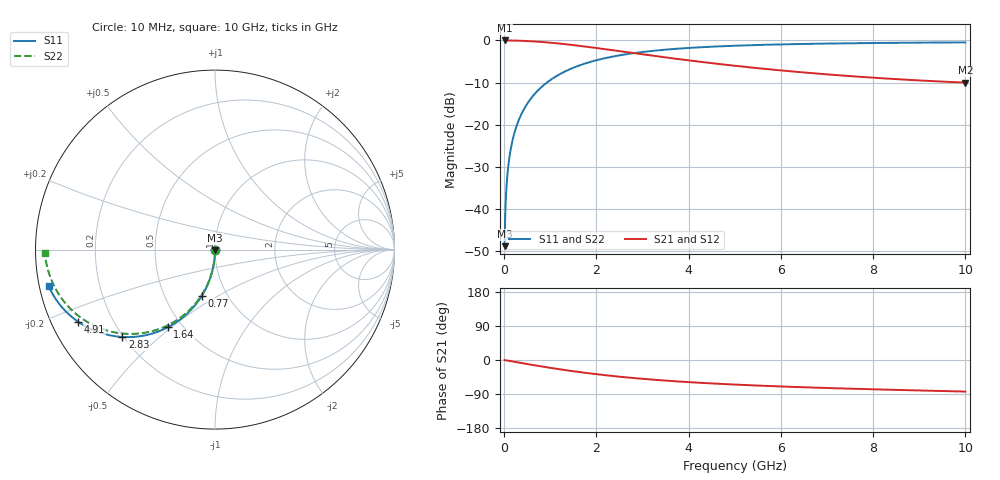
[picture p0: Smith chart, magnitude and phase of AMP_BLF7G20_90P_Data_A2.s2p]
! Created Tue May 08 13:45:06 2012
# ghz S ma R 50
! 2 Port Network Data from SP1.SP block
! freq  magS11  angS11  magS21  angS21  magS12  angS12  magS22  angS22
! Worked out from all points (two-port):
!   1000 points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, 10 MHz to 10 GHz, reference 50 ohm
!   highest |S21| = 0.00 dB at 10 MHz (marker M1); lowest = -10.0 dB at 10 GHz (marker M2)
!   |S21| within 3 dB of the highest: start of sweep to 2.804 GHz
!   lowest |S11| = -48.9 dB at 10 MHz (marker M3), VSWR 1.01, Z = 50 - j0.359 ohm
!   |S11| at or under -10 dB: start of sweep to 927.7 MHz
!   |S22| runs from -48.9 to -0.5 dB; largest |S21 - S12| = 0
!   S11 on the Smith chart (normalised r, x): 10 MHz: 1.00, -0.01; 770 MHz: 0.76, -0.42; 1.64 GHz: 0.42, -0.49; 2.83 GHz: 0.20, -0.38; 4.91 GHz: 0.08, -0.25; 10 GHz: 0.03, -0.11
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0.01  0.003594 -90.2  1 -0.2  1 -0.2  0.003594 -90.2
0.04  0.01438 -90.8  0.9999 -0.9  0.9999 -0.9  0.01438 -90.9
0.07  0.02516 -91.5  0.9997 -1.5  0.9997 -1.5  0.02516 -91.5
0.09  0.03234 -91.9  0.9995 -1.9  0.9995 -1.9  0.03234 -92.0
0.14  0.05028 -92.9  0.9987 -3.0  0.9987 -3.0  0.05028 -93.1
0.21  0.0753 -94.4  0.9971 -4.5  0.9971 -4.5  0.0753 -94.6
0.31  0.1108 -96.5  0.9938 -6.7  0.9938 -6.7  0.1108 -96.8
0.43  0.1528 -99.0  0.9882 -9.2  0.9882 -9.2  0.1528 -99.4
0.58  0.2041 -102.1  0.9789 -12.3  0.9789 -12.3  0.2041 -102.6
0.77  0.2667 -105.9  0.9637 -16.2  0.9637 -16.2  0.2667 -106.5
1.15  0.3817 -113.0  0.9243 -23.5  0.9243 -23.5  0.3817 -114.0
1.64  0.5068 -121.3  0.8621 -32.0  0.8621 -32.0  0.5067 -122.7
1.68  0.5158 -121.9  0.8567 -32.6  0.8567 -32.6  0.5158 -123.3
2.21  0.6197 -129.5  0.7848 -40.4  0.7848 -40.4  0.6197 -131.3
2.83  0.7093 -136.7  0.7048 -47.9  0.7048 -47.9  0.7093 -139.0
3.34  0.7634 -141.5  0.6459 -52.9  0.6459 -52.9  0.7634 -144.3
4.08  0.8197 -147.2  0.5727 -59.0  0.5727 -59.0  0.8197 -150.7
4.91  0.8621 -152.2  0.5067 -64.3  0.5067 -64.3  0.862 -156.4
5.01  0.8661 -152.7  0.4998 -64.9  0.4998 -64.9  0.8661 -157.1
6.67  0.9125 -159.6  0.409 -72.6  0.409 -72.6  0.9124 -165.7
8.34  0.9362 -164.3  0.3513 -78.4  0.3513 -78.4  0.9361 -172.5
10  0.9489 -167.7  0.3154 -83.4  0.3154 -83.4  0.9488 -178.9
